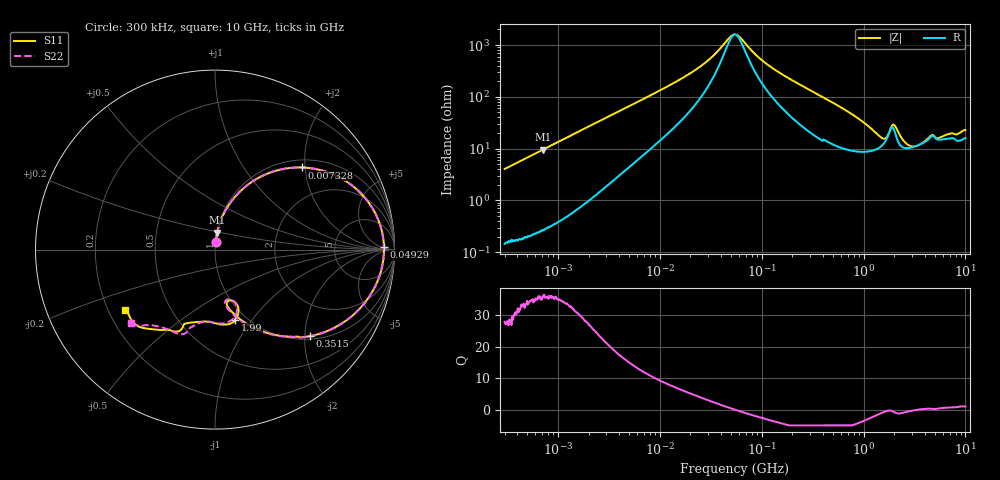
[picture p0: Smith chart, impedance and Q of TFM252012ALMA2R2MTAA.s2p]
! S-Parameter Data Generated by TDK Corporation
! Copyright(C) 2019 TDK Corporation.
! All Rights Reserved.
! TDK P/N: TFM252012ALMA2R2MTAA (Inductor)
! Property: L=2.2uH at 1MHz
! Size(LxWxT): 2.5x2x1.2mm
! Model Type: s2p (Touchstone File Format Version 1.0)
! Frequency: DC=Yes Start=0.3MHz Stop=10000MHz 802points Log-sweep
! Model Generated on May 10, 2019
! Port Assignments:
!  1 ---@@@--- 2
! Applicable Conditions:
!  Temperature = 25 degC
!  DC Bias Current = 0 A
!  Small Signal Operation
! Terms and conditions regarding TDK Simulation Models
! (1)This simulation model is being provided solely for informational purposes. Please refer to the specifications of the products in terms of detailed characteristics of such products.
! (2)In no event shall TDK Corporation of any of its subsidiaries be liable for any loss or damage arising, directly or indirectly,
!  From any information contained in this simulation model, including, but not limited to loss or damages arising from any inaccuracies, omissions or errors in connection with such information.
! (3)Any and all copyrights on this simulation model are owned by TDK Corporation.
!  Duplication or redistribution of this simulation model without prior written permission from TDK Corporation is prohibited.
! (4)This simulation model is subject to any modification or change without any prior notice.
! (5)Neither TDK Corporation nor any of its subsidiaries shall make any warranty, express or implied,
!  Including but not limited to the correctness, implied warranties of merchantability and fitness for a particular purpose with respect to this simulation models.
! (6)The use of this simulation model shall be deemed to have consented to the terms and conditions hereof.
# Hz S MA R 50
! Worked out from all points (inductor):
!   801 points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, 300 kHz to 10 GHz, reference 50 ohm
!   read as one part in series: L = 2.14 uH near 318.3 kHz
!   highest Q = 36 at 715.8 kHz (marker M1), where L = 2.13 uH
!   self-resonance near 54.85 MHz
!   S11 on the Smith chart (normalised r, x): 300 kHz: 1.00, +0.08; 7.328 MHz: 1.17, +1.93; 49.29 MHz: 31, +8; 351.5 MHz: 1.07, -2.12; 1.99 GHz: 0.89, -0.83; 10 GHz: 0.27, -0.28
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300000  0.04047 85.8  0.9977 -2.3  0.9975 -2.3  0.04059 85.8
715804  0.09527 83.0  0.993 -5.5  0.9927 -5.5  0.09529 82.9
1713600  0.2213 75.3  0.9678 -12.8  0.9676 -12.8  0.2213 75.3
3509086  0.4136 62.6  0.8891 -24.4  0.8891 -24.4  0.4135 62.6
7328194  0.6667 43.3  0.6901 -41.7  0.6902 -41.7  0.6666 43.3
9671944  0.7509 35.5  0.5866 -48.5  0.5866 -48.5  0.7508 35.5
2.504582e7  0.9152 12.9  0.2365 -62.9  0.2366 -62.9  0.915 12.8
4.929468e7  0.9415 0.9  0.06503 -25.6  0.06504 -25.6  0.9413 0.9
5.477226e7  0.9413 -0.8  0.05872 -1.2  0.05873 -1.2  0.9412 -0.9
1.210198e8  0.9079 -14.8  0.2337 58.6  0.2337 58.6  0.908 -14.9
3.126428e8  0.748 -38.8  0.5638 42.8  0.5638 42.8  0.7482 -39.0
3.514851e8  0.7153 -42.4  0.6059 39.5  0.6058 39.5  0.7156 -42.5
5.663179e8  0.5622 -56.7  0.748 25.0  0.748 25.0  0.5628 -56.9
9.101824e8  0.4173 -69.7  0.8354 9.9  0.8354 9.9  0.4185 -70.4
1.371335e9  0.324 -77.6  0.8596 -3.9  0.8596 -3.9  0.3215 -79.1
1.767019e9  0.303 -70.7  0.8015 -14.4  0.8015 -14.4  0.292 -72.5
1.990462e9  0.4053 -74.1  0.7424 -12.1  0.7424 -12.1  0.3963 -74.7
2.416286e9  0.4067 -91.8  0.8182 -16.3  0.8182 -16.3  0.4036 -93.3
3.303594e9  0.4178 -104.9  0.7997 -29.0  0.7997 -29.0  0.4211 -102.5
4.690952e9  0.4706 -112.6  0.7122 -43.1  0.7121 -43.2  0.4787 -108.4
6.899057e9  0.5613 -127.7  0.6437 -60.4  0.6437 -60.5  0.5508 -129.9
1e10  0.6059 -146.1  0.5468 -80.9  0.547 -81.0  0.6225 -139.0
